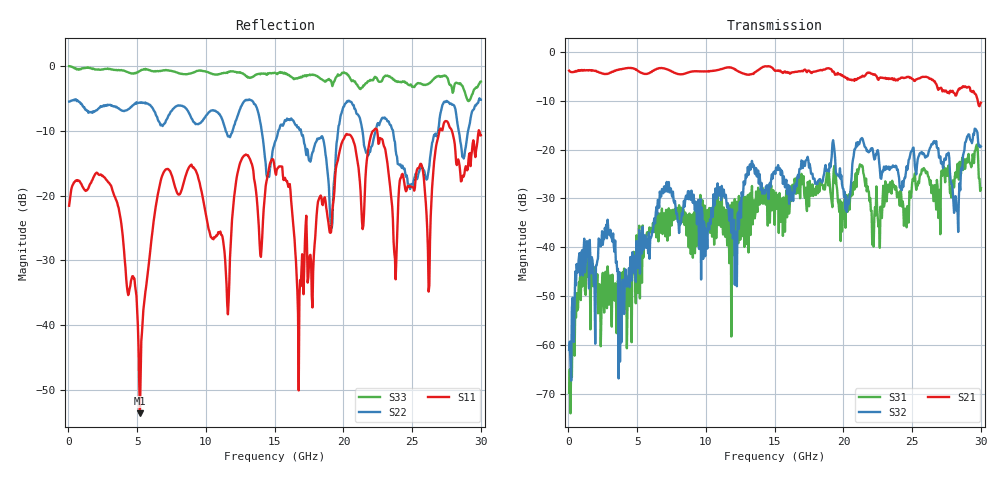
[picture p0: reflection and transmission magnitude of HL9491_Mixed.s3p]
! HYPERLABS, INC. 09/01/2021
! MIXED MODE  S-PARAMETERS
! CALCULATED FROM A MEASURED DATA S3P FILE
# GHZ S RI R 50.0
! FREQ.GHZ S11 SSD12 SSC12
! SDS21 SDD22 SDC22
! SCS21 SCD22 SCC22
!; PortSelection: Port_123
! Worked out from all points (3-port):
!   600 points, 50 MHz to 30 GHz, reference 50 ohm
!   strongest paths, dB at 50 MHz, 7.55 GHz, 15.05 GHz, 22.55 GHz, 30 GHz:
!     S21: -3.8, -4.1, -3.9, -5.7, -10.4
!     S32: -61.0, -29.7, -25.0, -20.9, -19.3
!     S31: -69.8, -33.9, -29.1, -35.8, -27.9
!   lowest |S11| = -53.7 dB at 5.2 GHz (marker M1), VSWR 1.00, Z = 50.2 - j0.00729 ohm
!   |S11| at or under -10 dB: start of sweep to 22.14 GHz; 22.46 GHz to 26.98 GHz (4.524 GHz wide, 18.3 % of centre); 27.9 GHz to 29.84 GHz (1.942 GHz wide, 6.73 % of centre)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
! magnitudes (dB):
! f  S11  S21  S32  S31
! 50 MHz  -21.6  -3.8  -61.0  -69.8
! 1 GHz  -18.5  -3.7  -40.6  -48.0
! 5.2 GHz  -53.7  -4.1  -45.4  -50.5
! 7 GHz  -16.1  -3.4  -27.5  -34.4
! 11.55 GHz  -36.8  -3.2  -31.9  -39.6
! 15.05 GHz  -16.4  -3.9  -25.0  -29.1
! 16.75 GHz  -50.1  -4.0  -25.7  -25.6
! 20.2 GHz  -10.5  -5.3  -29.6  -29.3
! 23.75 GHz  -29.8  -5.7  -23.6  -28.2
! 30 GHz  -10.7  -10.4  -19.3  -27.9
